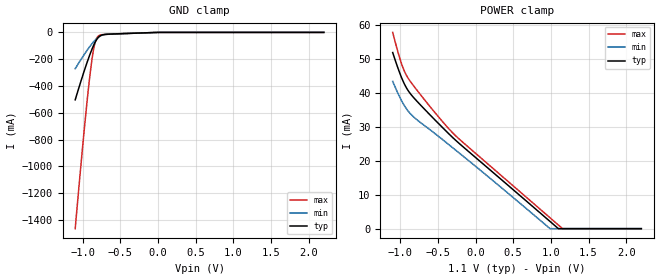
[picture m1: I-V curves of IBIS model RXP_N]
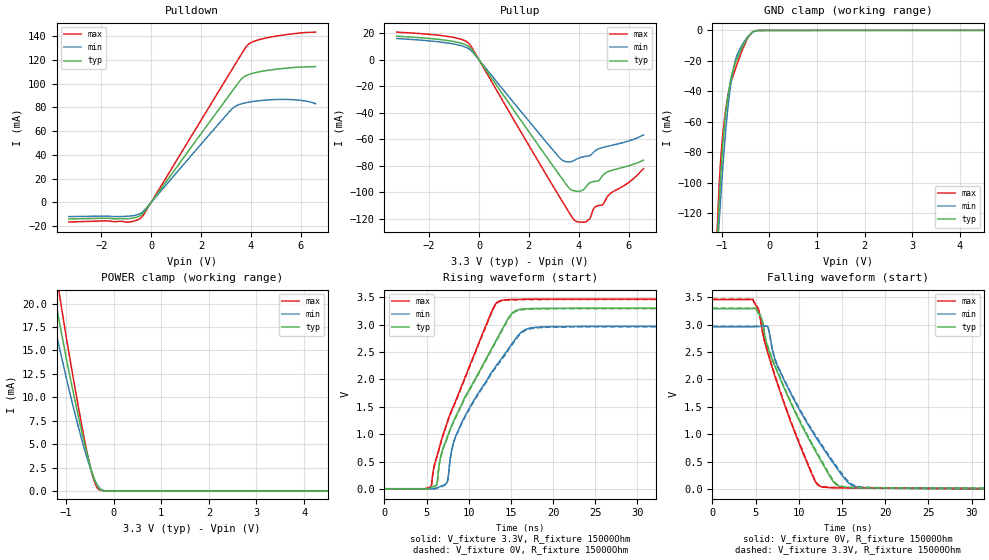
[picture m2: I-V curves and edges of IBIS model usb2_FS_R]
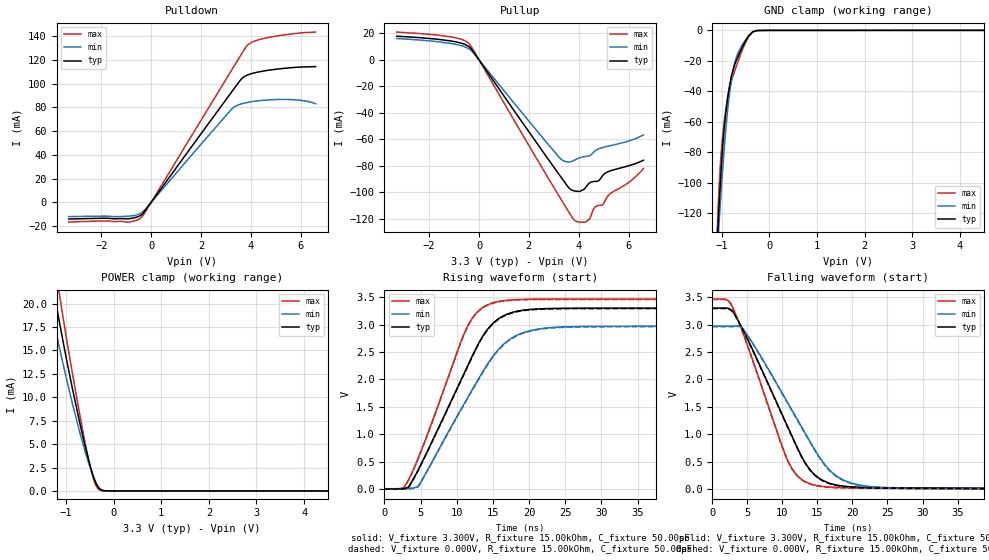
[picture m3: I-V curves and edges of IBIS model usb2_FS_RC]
| Texas Instruments Incorporated
| Four-Port USB 3.0 Hub
| Marketing part#   Voltage Range   Package-type   Temperature
| TUSB8041PAPQ1   2.97V - 3.465V   64-Pin HTQFP   -45 to 85 C
[IBIS Ver]   4.1
[File name]   tusb8041q1.ibs
[File Rev]   1.0
[Date]   02/28/2014
[Source]   Model built from TISPICE simulations at:
   Texas Instruments Incorporated.
   Analog-eLab, HPA
   12500 TI Blvd
   Dallas, TX -75243
[Notes]   Rev 1.0: 02/28/2014
   - Model based on v1.0 IBIS model for TUSB8040 dated 01/25/2012
   - Model generated from simulations in TISPICED
   - For USB2.0, models are included for HS, FS and LS modes
   - For USB3.0, models are included for No-De-Emphasis and De-Emphasis modes
   - USB2 and USB3 Models  matched to TISPICE.
   - C_comp although listed in numerical order of value are obtained from varying
   PVT conditions. For PVT conditions for each specific value refer the buffer
   description under respective [Model]. IBIS model user is responsible for using
   appropriate C_comp to simulate for Signal Integrity
   Where for TUSB8041
   Nom PVT:  Nominal process, Typ Temperature, Typ Voltage
   Slow PVT: Weak process, Max Temperature, Min Voltage
   Fast PVT: Strong process, Min Temperatire, Max Voltage
   - ignore warnings related to usb3_WODE, please do not correct this error
   as IBIS parser does not correct IV-VT mismatch with single set of V-T
   waveforms.
   - non-monotonic warnings related to usb2_LS_RC and usb2_LS_R buffers are
   as they are seen in TISPICE simualations
   - [Driver Schedule] is interpreted differently by each system level simulator
   , if usual setup with it does not give appropriate results, please
   tie the MAIN and BOOST buffers as per buffer timing description under
   [Driver Schedule] keyword. For example, using HSPICE, refer DE_hspice.sp
   in the correlation report
   - To test USB2/USB3 IBIS models using HSPICE look for spice set up files
   inside the TUSB8040 correlation report   \
   - Non-Monotonic pulldown warnings related to digital buffers is per
   simulations
[Disclaimer] This product is designed as an aid for customers of Texas Instruments.
   No warranties, either expressed or implied, with respect to this third
   party software (if any) or with respect to its fitness for any
   particular purpose is claimed by Texas Instruments or the author. The
   software (if any) is provided solely on an "as is" basis. The entire
   risk as to its quality and performance is with the customer
[Copyright]   (C)Copyright 2014 Texas Instruments Incorporated.
   All rights reserved.
|   TUSB8041
[Component]   TUSB8041
[Manufacturer]  Texas Instruments Incorporated
[Package]   |64-pin HTQFP
|   typ   min   max
R_pkg   0.2389   0.0142   0.3346
L_pkg   2.3741nH   1.4298nH   2.8522nH
C_pkg   0.8499pF   0.7143pF   1.0609pF
[PIN]   signal_name   model_name   R_pin   L_pin   C_pin
1   PWRCTL3/BATEN3   FZP18_PD_PI_10P_3P3   NA   NA   NA
2   VDD33   POWER   NA   NA   NA
3   PWRCTL2/BATEN2   FZP18_PD_PI_10P_3P3   NA   NA   NA
4   PWRCTL1/BATEN1   FZP18_PD_PI_10P_3P3   NA   NA   NA
5   SDA/SMBDAT   FZP18_PD_PI_10P_3P3   NA   NA   NA
6   SCL/SMBCLK   FZP18_PD_PI_10P_3P3   NA   NA   NA
7   SMBUSZ/SS_SUSPEND   FZP18_PU_PI_10P_3P3   NA   NA   NA
8   FULLPWRMGMT   FZP18_PD_PI_10P_3P3   NA   NA   NA
9   POWCTL_POL   FZP18_PU_PI_10P_3P3   NA   NA   NA
10   GANGED/SMBAS2   FZP18_PD_PI_10P_3P3   NA   NA   NA
11   OVERCUR4Z   PBFZP18_PU_10P   NA   NA   NA
12   OVERCUR3Z   PBFZP18_PU_10P   NA   NA   NA
13   AUTOENZ/HS_SUSPEND   FZP18_PU_PI_10P_3P3   NA   NA   NA
14   OVERCUR1Z   PBFZP18_PU_10P   NA   NA   NA
15   OVERCUR2Z   PBFZP18_PU_10P   NA   NA   NA
16   USB_VBUS   C33SHYPBFZP18_10P   NA   NA   NA
17   TEST   YPBFZP18_PD_10P   NA   NA   NA
18   GRSTZ   PBFZP18_PU_10P   NA   NA   NA
19   VDD   POWER   NA   NA   NA
20   VDD33   POWER   NA   NA   NA
21   USB_DP_UP   usb2   NA   NA   NA
22   USB_DM_UP   usb2   NA   NA   NA
23   USB_SSTXP_UP   usb3   NA   NA   NA
24   USB_SSTXM_UP   usb3   NA   NA   NA
25   VDD   POWER   NA   NA   NA
26   USB_SSRXP_UP   RXP_N   NA   NA   NA
27   USB_SSRXM_UP   RXP_N   NA   NA   NA
28   NC   NC   NA   NA   NA
29   XO   NC   NA   NA   NA
30   XI   NC   NA   NA   NA
31   VDD33   POWER   NA   NA   NA
32   USB_R1   NC   NA   NA   NA
33   USB_DP_DN1   usb2   NA   NA   NA
34   USB_DM_DN1   usb2   NA   NA   NA
35   USB_SSTXP_DN1   usb3   NA   NA   NA
36   USB_SSTXM_DN1   usb3   NA   NA   NA
37   VDD   POWER   NA   NA   NA
38   USB_SSRXP_DN1   RXP_N   NA   NA   NA
39   USB_SSRXM_DN1   RXP_N   NA   NA   NA
40   NC   NC   NA   NA   NA
41   USB_DP_DN2   usb2   NA   NA   NA
42   USB_DM_DN2   usb2   NA   NA   NA
43   USB_SSTXP_DN2   usb3   NA   NA   NA
44   USB_SSTXM_DN2   usb3   NA   NA   NA
45   VDD   POWER   NA   NA   NA
46   USB_SSRXP_DN2   RXP_N   NA   NA   NA
47   USB_SSRXM_DN2   RXP_N   NA   NA   NA
48   VDD33   POWER   NA   NA   NA
49   USB_DP_DN3   usb2   NA   NA   NA
50   USB_DM_DN3   usb2   NA   NA   NA
51   USB_SSTXP_DN3   usb3   NA   NA   NA
52   USB_SSTXM_DN3   usb3   NA   NA   NA
53   VDD   POWER   NA   NA   NA
54   USB_SSRXP_DN3   RXP_N   NA   NA   NA
55   USB_SSRXM_DN3   RXP_N   NA   NA   NA
56   USB_DP_DN4   usb2   NA   NA   NA
57   USB_DM_DN4   usb2   NA   NA   NA
58   USB_SSTXP_DN4   usb3   NA   NA   NA
59   USB_SSTXM_DN4   usb3   NA   NA   NA
60   VDD   POWER   NA   NA   NA
61   USB_SSRXP_DN4   RXP_N   NA   NA   NA
62   USB_SSRXM_DN4   RXP_N   NA   NA   NA
63   VDD   POWER   NA   NA   NA
64   PWRCTL4/BATEN4   FZP18_PD_PI_10P_3P3   NA   NA   NA
[Diff_pin]   inv_pin   vdiff   tdelay_typ   tdelay_min   tdelay_max
23   24   NA   NA   NA   NA
26   27   200mV   NA   NA   NA
21   22   NA   NA   NA   NA
35   36   NA   NA   NA   NA
38   39   200mV   NA   NA   NA
33   34   NA   NA   NA   NA
43   44   NA   NA   NA   NA
46   47   200mV   NA   NA   NA
41   42   NA   NA   NA   NA
51   52   NA   NA   NA   NA
54   55   200mV   NA   NA   NA
49   50   NA   NA   NA   NA
58   59   NA   NA   NA   NA
61   62   200mV   NA   NA   NA
56   57   NA   NA   NA   NA
[Model Selector] usb2
usb2_HS_R   USB 2.0 High Speed mode, for DP/DM pin 240MHz
usb2_HS_RC   USB 2.0 High Speed mode, for DP/DM pin 240MHz, with Cfixture
usb2_FS_R   USB 2.0 Fast Speed mode, for DP/DM pin 6MHz
usb2_FS_RC   USB 2.0 Fast Speed mode, for DP/DM pin 6MHz, with Cfixture
usb2_LS_RC   USB 2.0 Low  Speed mode, for DP/DM pin 750kHz, with Cfixture
usb2_LS_R   USB 2.0 Low  Speed mode, for DP/DM pin 750kHz
[Model Selector] usb3
usb3_DE   USB 3.0 De-Emphasis mode, best at 1.25GHz
usb3_WODE   USB 3.0 No De-Emphasis mode, for SSTXP/N 2.5GHz
|USB 3.0 De-Emphasis mode, for SSTXP/SSTXN pins 2.5Gbps(1.25GHz to De-Emphasis)
[Model]   usb3_DE
Model_type   Output
Vmeas = 1.1
Vref = 1.1
Rref = 50
|   typ   min   max
|   (TYP PVT)   (Fast PVT) (Slow PVT)
C_comp   0pF   0pF   0pF
[Driver Schedule]
| Model_name   Rise_on_dly Rise_off_dly Fall_on_dly Fall_off_dly
usb3_de_MAIN   0.0nS   NA   0   NA
usb3_de_BOOST   NA   0.2nS   NA   0.2nS
[Voltage Range]   1.1   0.99   1.155
[Temperature Range]   27   105   -40
[Pullup Reference]   1.1   0.99   1.155
[Pulldown Reference]   0   0   0
[Power Clamp Reference]   1.1   0.99   1.155
[GND Clamp Reference]   0   0   0
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[Ramp]
R_load = 50
|   typ   min   max
dV/dt_r   0.972315/1.549e-011   0.988218/1.8606e-011   0.957162/1.40763e-011
dV/dt_f   0.972312/7.7916e-012   0.988183/1.21282e-011  0.957081/6.00194e-012
| Models and submodels in the file (16): RXP_N (Input), usb2_FS_R (I/O), usb2_FS_RC (I/O), usb2_HS_R (I/O), usb2_HS_RC (I/O), usb2_LS_R (I/O), usb2_LS_RC (I/O), usb3_WODE (Output), usb3_DE (Output), usb3_de_MAIN (Output), usb3_de_BOOST (Open_drain), FZP18_PD_PI_10P_3P3 (I/O), YPBFZP18_PD_10P (Input), PBFZP18_PU_10P (Input), C33SHYPBFZP18_10P (Input), FZP18_PU_PI_10P_3P3 (I/O)
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|   RXP_N Input model
[Model]   RXP_N
Model_type   Input
Vinl = 0.35V
Vinh = 0.715V
|   typ   min   max
|   (nom PVT)   (Fast PVT)   (slow PVT)
C_comp   2.352pF   1.988pF   2.902pF
[Voltage Range]   1.1   0.99   1.155
[Temperature Range]   27   105   -40
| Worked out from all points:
|   GND clamp passes 1 mA (typ) near -0.05 V on its own axis
[GND Clamp]
|   Voltage   I(typ)   I(min)   I(max)
-1.1V     -503.3mA   -270.9mA   -1.465A
-1.034V   -381.9mA   -211.2mA   -1.049A
-984.2mV  -294.5mA   -168.2mA   -750.8mA
-942.9mV  -225mA     -134mA     -516.7mA
-901.5mV  -160mA     -101.8mA   -306.1mA
-868.4mV  -113.2mA   -78.33mA   -167.8mA
-843.6mV  -82.41mA   -62.44mA   -92.88mA
-818.8mV  -56.94mA   -48.5mA    -48.05mA
-794mV    -38.04mA   -36.95mA   -27.66mA
-694.7mV  -14.71mA   -15.15mA   -14.99mA
0V        0A         0A         0A
2.2V      0A         0A         0A
[POWER Clamp]
|   Voltage   I(typ)   I(min)   I(max)
-1.1V     51.96mA    43.46mA    57.9mA
-1.042V   48.11mA    40.5mA     53.03mA
-992.5mV  45.12mA    38.19mA    49.32mA
-951.1mV  42.97mA    36.52mA    46.79mA
-909.8mV  41.25mA    35.11mA    44.92mA
-794mV    37.98mA    32.41mA    41.31mA
-421.8mV  29.45mA    25.99mA    31.15mA
-198.5mV  24.77mA    21.98mA    26.05mA
984.2mV   2.206mA    77.67uA    3.283mA
1.1V      0A         0A         1.052mA
1.15V     0A         0A         96.58uA
2.2V      0A         0A         0A
|   USB 2.0 Fast Speed mode, for DP pin 6MHz
[Model]   usb2_FS_R
Model_type   I/O
Polarity   Non-Inverting
Enable   Active-High
Vmeas = 1.54
Vref = 0
Rref = 15000
Cref = 50pF
Vinl = 0.8V
Vinh = 2.0V
|   typ   min   max
|   (nom PVT)   (Fast PVT)   (slow PVT)
C_comp   9.0376pF   8.9385pF   9.1512pF
[Voltage Range]   3.3   2.97   3.465
[Temperature Range]   27   105   -40
[Pullup Reference]   3.3   2.97   3.465
[Pulldown Reference]   -0   -0   -0
[Power Clamp Reference]   3.3   2.97   3.465
[GND Clamp Reference]   -0   -0   -0
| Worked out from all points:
|   slope of the pulldown table from 0 to 0.495 V, typ, clamps not added: 34.6 ohm
|   slope of the pullup table from 0 to 0.495 V, typ, clamps not added: 36.8 ohm
|   GND clamp passes 1 mA (typ) near -0.35 V on its own axis
|   POWER clamp passes 1 mA (typ) near -0.39 V on its own axis
|   falling waveform, V_fixture 0V, R_fixture 15000Ohm: 20-80 % time 5.73ns typ, 6.23ns min, 4.47ns max; typ from 3.29 V to 0 V
|   rising waveform, V_fixture 3.3V, R_fixture 15000Ohm: 20-80 % time 6.21ns typ, 6.02ns min, 5.07ns max; typ from 0.008 V to 3.3 V
|   rising waveform, V_fixture 0V, R_fixture 15000Ohm: 20-80 % time 6.24ns typ, 6.08ns min, 5.09ns max; typ from 0 V to 3.29 V
|   falling waveform, V_fixture 3.3V, R_fixture 15000Ohm: 20-80 % time 5.77ns typ, 6.3ns min, 4.5ns max; typ from 3.3 V to 0.008 V
[Pulldown]
|   Voltage   I(typ)   I(min)   I(max)
-3.3V     -13.97mA   -11.94mA   -16.5mA
-1.865V   -13.31mA   -11.55mA   -15.58mA
-948.8mV  -13.78mA   -11.64mA   -16.64mA
-429mV    -11.05mA   -9.328mA   -13.36mA
-255.8mV  -7.37mA    -6.247mA   -8.827mA
3.234V    93.1mA     78.54mA    111.5mA
3.61V     103.6mA    82.92mA    124.4mA
3.858V    107.2mA    84.17mA    132.2mA
4.15V     109.1mA    85.16mA    135.8mA
4.714V    111.3mA    86.32mA    138.9mA
5.798V    113.7mA    86.37mA    142.3mA
6.6V      114.4mA    83.14mA    143.4mA
[GND Clamp]
|   Voltage   I(typ)   I(min)   I(max)
-3.3V     -2.986A    -2.594A    -3.408A
-1.102V   -142.8mA   -148.5mA   -133.6mA
-1.068V   -120.4mA   -130.9mA   -108.6mA
-1.053V   -111.5mA   -123.5mA   -99.43mA
-1.028V   -97.72mA   -111.6mA   -86.34mA
-948.8mV  -63.66mA   -76.9mA    -59.29mA
-874.5mV  -43.76mA   -51.14mA   -43.02mA
-795.3mV  -29.32mA   -31.84mA   -32.77mA
-676.5mV  -18.29mA   -15.93mA   -21.75mA
-458.7mV  -4.679mA   -4.168mA   -5.163mA
-349.8mV  -954.6uA   -1.019mA   -868.7uA
6.6V      27.44uA    21.44uA    34.47uA
[Pullup]
|   Voltage   I(typ)   I(min)   I(max)
-3.3V     17.86mA    16.11mA    20.95mA
-1.162V   14.34mA    12.44mA    17.42mA
-374.6mV  9.504mA    7.922mA    11.72mA
3.224V    -86.72mA   -73.66mA   -103.1mA
3.625V    -96.87mA   -77.02mA   -115.4mA
3.863V    -98.94mA   -75.34mA   -121.4mA
4.303V    -95.54mA   -72.68mA   -122mA
4.452V    -92.62mA   -72.08mA   -119.5mA
4.655V    -91.65mA   -68.64mA   -111mA
4.962V    -87.23mA   -66.09mA   -109.1mA
5.14V     -84.63mA   -65.26mA   -103.4mA
6.6V      -75.66mA   -56.61mA   -82.01mA
[POWER Clamp]
|   Voltage   I(typ)   I(min)   I(max)
-3.3V     96.11mA    80.39mA    114.3mA
-1.409V   25.5mA     21.48mA    30.05mA
-1.315V   22.86mA    19.29mA    26.86mA
-1.246V   20.93mA    17.7mA     24.52mA
-1.127V   17.68mA    15mA       20.59mA
-854.7mV  10.64mA    9.089mA    12.22mA
-567.6mV  4.132mA    3.664mA    4.338mA
-419.1mV  1.439mA    1.425mA    1.205mA
-359.7mV  684.8uA    768.2uA    455.6uA
-290.4mV  187uA      273.4uA    86.97uA
0V        0A         0A         0A
6.6V      0A         0A         0A
[Ramp]
R_load = 15000
|   typ   min   max
dV/dt_r   1.97481/6.20846e-009   1.77621/6.02152e-009   2.07437/5.07374e-009
dV/dt_f   1.97455/5.7255e-009   1.77598/6.2317e-009   2.07413/4.47102e-009
[Falling Waveform]
V_fixture = 0V
V_fixture_min = 0V
V_fixture_max = 0V
R_fixture = 15000Ohm
C_fixture = 0F
|   Time   V(typ)   V(min)   V(max)
0s        3.291V     2.961V     3.457V
4.7ns     3.293V     2.961V     3.458V
5.7ns     3.108V     2.967V     2.957V
6.4ns     2.601V     2.967V     2.494V
7.5ns     2.143V     2.254V     1.936V
11.4ns    846.1mV    1.091V     316.1mV
12.6ns    506.4mV    796.2mV    44.4mV
14.4ns    75.51mV    384.1mV    24.24mV
17.5ns    21.5mV     25.98mV    19.1mV
84.9ns    94.35uV    653.8uV    37.35uV
[Rising Waveform]
|Vcc
V_fixture = 3.3V
V_fixture_min = 2.97V
V_fixture_max = 3.465V
R_fixture = 15000Ohm
C_fixture = 0F
|   Time   V(typ)   V(min)   V(max)
0s        7.658mV    8.716mV    6.679mV
5.5ns     34.03mV    9.217mV    46.24mV
6.2ns     85.76mV    22.01mV    590.8mV
6.6ns     542.7mV    47.18mV    807.5mV
7.4ns     926.5mV    115.1mV    1.193V
8.6ns     1.371V     1.019V     1.668V
13.8ns    2.867V     2.361V     3.438V
15.3ns    3.227V     2.686V     3.457V
18.1ns    3.293V     2.951V     3.462V
84.9ns    3.299V     2.969V     3.464V
[Rising Waveform]
V_fixture = 0V
V_fixture_min = 0V
V_fixture_max = 0V
R_fixture = 15000Ohm
C_fixture = 0F
|   Time   V(typ)   V(min)   V(max)
0s        100.2uV    720.6uV    39.4uV
5.5ns     26.33mV    1.222mV    39.41mV
6.2ns     77.72mV    13.9mV     579.6mV
6.6ns     530.5mV    39.01mV    795.4mV
7.4ns     911.9mV    106.6mV    1.179V
8.6ns     1.353V     1.003V     1.653V
13.8ns    2.848V     2.339V     3.429V
15.5ns    3.233V     2.707V     3.45V
18.3ns    3.285V     2.942V     3.455V
84.9ns    3.291V     2.961V     3.457V
[Falling Waveform]
|Gnd
V_fixture = 3.3V
V_fixture_min = 2.97V
V_fixture_max = 3.465V
R_fixture = 15000Ohm
C_fixture = 0F
|   Time   V(typ)   V(min)   V(max)
0s        3.299V     2.969V     3.464V
4.7ns     3.301V     2.97V      3.465V
5.7ns     3.117V     2.975V     2.966V
6.4ns     2.614V     2.976V     2.506V
7.5ns     2.159V     2.27V      1.952V
11.5ns    841mV      1.091V     299.3mV
12.7ns    502.5mV    798.8mV    49.57mV
14.4ns    91.03mV    411.2mV    31.27mV
17.6ns    29.38mV    35.57mV    25.66mV
84.9ns    7.652mV    8.648mV    6.677mV
|   USB 2.0 Fast Speed mode, for DM pin 6MHz with recommended C load of 50pF.
[Model]   usb2_FS_RC
Model_type   I/O
Polarity   Non-Inverting
Enable   Active-High
Vmeas = 1.54
Vref = 0
Rref = 15000
Cref = 50pF
Vinl = 0.8V
Vinh = 2.0V
|   typ   min   max
|   (nom PVT)   (Fast PVT)   (slow PVT)
C_comp   9.0376pF   8.9385pF   9.1512pF
[Voltage Range]   3.3   2.97   3.465
[Temperature Range]   27   105   -40
[Pullup Reference]   3.3   2.97   3.465
[Pulldown Reference]   -0   -0   -0
[Power Clamp Reference]   3.3   2.97   3.465
[GND Clamp Reference]   -0   -0   -0
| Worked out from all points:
|   slope of the pulldown table from 0 to 0.495 V, typ, clamps not added: 34.6 ohm
|   slope of the pullup table from 0 to 0.495 V, typ, clamps not added: 36.8 ohm
|   GND clamp passes 1 mA (typ) near -0.35 V on its own axis
|   POWER clamp passes 1 mA (typ) near -0.39 V on its own axis
|   falling waveform, V_fixture 3.300V, R_fixture 15.00kOhm, C_fixture 50.00pF: 20-80 % time 7.09ns typ, 8.08ns min, 5.62ns max; typ from 3.3 V to 0.008 V
|   rising waveform, V_fixture 3.300V, R_fixture 15.00kOhm, C_fixture 50.00pF: 20-80 % time 7.12ns typ, 7.76ns min, 5.77ns max; typ from 0.008 V to 3.3 V
|   rising waveform, V_fixture 0.000V, R_fixture 15.00kOhm, C_fixture 50.00pF: 20-80 % time 7.12ns typ, 7.77ns min, 5.77ns max; typ from 0 V to 3.29 V
|   falling waveform, V_fixture 0.000V, R_fixture 15.00kOhm, C_fixture 50.00pF: 20-80 % time 7.08ns typ, 8.07ns min, 5.61ns max; typ from 3.29 V to 0 V
[Pulldown]
|   Voltage   I(typ)   I(min)   I(max)
-3.3V     -13.97mA   -11.94mA   -16.5mA
-1.865V   -13.31mA   -11.55mA   -15.58mA
-948.8mV  -13.78mA   -11.64mA   -16.64mA
-429mV    -11.05mA   -9.328mA   -13.36mA
-255.8mV  -7.37mA    -6.247mA   -8.827mA
3.234V    93.1mA     78.54mA    111.5mA
3.61V     103.6mA    82.92mA    124.4mA
3.858V    107.2mA    84.17mA    132.2mA
4.15V     109.1mA    85.16mA    135.8mA
4.714V    111.3mA    86.32mA    138.9mA
5.798V    113.7mA    86.37mA    142.3mA
6.6V      114.4mA    83.14mA    143.4mA
[GND Clamp]
|   Voltage   I(typ)   I(min)   I(max)
-3.3V     -2.986A    -2.594A    -3.408A
-1.102V   -142.8mA   -148.5mA   -133.6mA
-1.068V   -120.4mA   -130.9mA   -108.6mA
-1.053V   -111.5mA   -123.5mA   -99.43mA
-1.028V   -97.72mA   -111.6mA   -86.34mA
-948.8mV  -63.66mA   -76.9mA    -59.29mA
-874.5mV  -43.76mA   -51.14mA   -43.02mA
-795.3mV  -29.32mA   -31.84mA   -32.77mA
-676.5mV  -18.29mA   -15.93mA   -21.75mA
-458.7mV  -4.679mA   -4.168mA   -5.163mA
-349.8mV  -954.6uA   -1.019mA   -868.7uA
6.6V      27.44uA    21.44uA    34.47uA
[Pullup]
|   Voltage   I(typ)   I(min)   I(max)
-3.3V     17.86mA    16.11mA    20.95mA
-1.162V   14.34mA    12.44mA    17.42mA
-374.6mV  9.504mA    7.922mA    11.72mA
3.224V    -86.72mA   -73.66mA   -103.1mA
3.625V    -96.87mA   -77.02mA   -115.4mA
3.863V    -98.94mA   -75.34mA   -121.4mA
4.303V    -95.54mA   -72.68mA   -122mA
4.452V    -92.62mA   -72.08mA   -119.5mA
4.655V    -91.65mA   -68.64mA   -111mA
4.962V    -87.23mA   -66.09mA   -109.1mA
5.14V     -84.63mA   -65.26mA   -103.4mA
6.6V      -75.66mA   -56.61mA   -82.01mA
[POWER Clamp]
|   Voltage   I(typ)   I(min)   I(max)
-3.3V     96.11mA    80.39mA    114.3mA
-1.409V   25.5mA     21.48mA    30.05mA
-1.315V   22.86mA    19.29mA    26.86mA
-1.246V   20.93mA    17.7mA     24.52mA
-1.127V   17.68mA    15mA       20.59mA
-854.7mV  10.64mA    9.089mA    12.22mA
-567.6mV  4.132mA    3.664mA    4.338mA
-419.1mV  1.439mA    1.425mA    1.205mA
-359.7mV  684.8uA    768.2uA    455.6uA
-290.4mV  187uA      273.4uA    86.97uA
0V        0A         0A         0A
6.6V      0A         0A         0A
[Ramp]
R_load = 15.00kOhm
|   typ   min   max
dV/dt_r   1.975V/7.118ns   1.776V/7.768ns   2.074V/5.764ns
dV/dt_f   1.975V/7.089ns   1.777V/8.081ns   2.074V/5.614ns
[Falling Waveform]
V_fixture = 3.300V
V_fixture_min = 2.970V
V_fixture_max = 3.465V
R_fixture = 15.00kOhm
C_fixture = 50.00pF
|   Time   V(typ)   V(min)   V(max)
0s        3.299V     2.969V     3.464V
2.4ns     3.286V     2.97V      3.419V
4.2ns     2.947V     2.947V     2.907V
10.69ns   1.157V     1.59V      545mV
12.14ns   753.6mV    1.267V     246.5mV
14.07ns   335.9mV    840.6mV    94.42mV
15.85ns   154.3mV    481.3mV    48.71mV
17.64ns   77.37mV    248.2mV    32.68mV
22.25ns   29.92mV    52.16mV    21.45mV
83.29ns   7.582mV    8.019mV    6.667mV
[Rising Waveform]
V_fixture = 3.300V
V_fixture_min = 2.970V
V_fixture_max = 3.465V
R_fixture = 15.00kOhm
C_fixture = 50.00pF
|   Time   V(typ)   V(min)   V(max)
0s        7.582mV    8.019mV    6.667mV
2.63ns    14.86mV    8.107mV    23.09mV
3.35ns    42.86mV    10.65mV    176.9mV
4.68ns    354.6mV    57.1mV     571.4mV
11.34ns   2.202V     1.63V      2.927V
12.88ns   2.621V     1.981V     3.234V
14.9ns    3.01V      2.403V     3.391V
18.36ns   3.243V     2.808V     3.454V
23.8ns    3.294V     2.952V     3.463V
83.29ns   3.299V     2.969V     3.464V
[Rising Waveform]
V_fixture = 0.000V
V_fixture_min = 0.000V
V_fixture_max = 0.000V
R_fixture = 15.00kOhm
C_fixture = 50.00pF
|   Time   V(typ)   V(min)   V(max)
0s        3.197uV    8.923uV    4.349uV
2.63ns    7.278mV    96.94uV    16.39mV
3.36ns    36.84mV    2.771mV    171.8mV
4.68ns    345.4mV    48.95mV    562.8mV
11.35ns   2.193V     1.621V     2.921V
12.89ns   2.613V     1.97V      3.227V
14.91ns   3.001V     2.393V     3.384V
18.18ns   3.229V     2.786V     3.446V
23.01ns   3.284V     2.936V     3.456V
83.29ns   3.291V     2.961V     3.457V
[Falling Waveform]
V_fixture = 0.000V
V_fixture_min = 0.000V
V_fixture_max = 0.000V
R_fixture = 15.00kOhm
C_fixture = 50.00pF
|   Time   V(typ)   V(min)   V(max)
0s        3.291V     2.961V     3.457V
2.4ns     3.278V     2.961V     3.412V
4.2ns     2.937V     2.938V     2.898V
10.67ns   1.15V      1.581V     540.7mV
12.12ns   746.6mV    1.258V     240.7mV
14.05ns   328.3mV    831mV      87.96mV
15.83ns   146.5mV    471.7mV    42.08mV
17.61ns   69.9mV     239.9mV    26.07mV
22.23ns   22.29mV    43.83mV    14.8mV
83.29ns   3.197uV    8.923uV    4.349uV
